[IBIS ver]   4.2
[File name]   tm4c123gh6pge_144qfp_v0p0.ibs
[File Rev]   v0p0
[Date]   Oct 16, 2013
[Source]   simulation
[Notes]   IBIS models for 144qfp package with updated GPIO models
[Disclaimer] Please be aware that in the absence of a written agreement,
   Texas Instruments (TI) assumes no liability for: 1) the
   accuracy of the IBIS models provided to your company, 2) the
   proper functioning of these IBIS models in your design or for
   any resulting applications, or; 3) infringement of patents,
   copyrights, or intellectual property rights resulting from
   your use of these IBIS models. TI provides IBIS models as a
   service to our customers and therefore reserves the right to
   limit distribution of the IBIS models.
   This preliminary model does not contain all of the possible pad
   models for each of the pad types.  The most commonly used modes
   have been provided and the next update will include all of the
   pad model combinations.
   The only missing model that needs to be highlighted is the
   model for the USB D+ and D- GPIOs.  Currently only the USB
   functionality is provided on the D+ and D- pins.  Customers
   needing to model the PGIOs associated with these pins should
   check for a newer model.
[Copyright]   Property of Texas Instruments Incorporated. Unauthorized
   reproduction and/or distribution is strictly prohibited. This
   product is protected under copyright law and trade secret law
   as an unpublished work. Copyright (C) 2013, Texas Instruments
   Incorporated, all rights reserved. These commodities are under
   the U.S. Government distribution license control. As such,
   they are not to be re-exported without the prior approval of
   the U.S. Department of Commerce.
|   Component TM4C123GH6PGE
[Component]   TM4C123GH6PGE
[Manufacturer]   Texas Instruments Inc.
[Package]
| 144-pin QFP
| variable   typ   min   max
R_Pkg   2.69E-01   2.45E-01   3.00E-01
L_pkg   7.59E-09   5.97E-09   9.02E-09
C_pkg   1.89E-12   1.71E-12   2.18E-12
[Pin]   signal_name   model_name   R_pin   L_pin   C_pin
1   PD0   GPIO8P_5V   2.98E-01   8.84E-09   1.79E-12
2   PD1   GPIO8P_5V   2.91E-01   8.75E-09   2.17E-12
3   PD2   GPIO8P_5V   2.87E-01   8.56E-09   2.13E-12
4   PD3   GPIO8P_5V   2.79E-01   8.34E-09   2.08E-12
5   VDD   POWER
6   GND   GND
7   VDDA   POWER
8   VREFAP   NC
9   VREFAM   NC
10   GNDA   GND
11   PP2   GPIO8P_5V   2.64E-01   7.47E-09   1.85E-12
12   PE3   GPIO8P_5V   2.60E-01   7.38E-09   1.83E-12
13   PE2   GPIO8P_5V   2.54E-01   7.11E-09   1.81E-12
14   PE1   GPIO8P_5V   2.53E-01   6.97E-09   1.78E-12
15   PE0   GPIO8P_5V   2.49E-01   6.94E-09   1.74E-12
16   PK0   GPIO8P_5V   2.50E-01   6.88E-09   1.72E-12
17   PK1   GPIO8P_5V   2.48E-01   6.76E-09   1.72E-12
18   PK2   GPIO8P_5V   2.48E-01   6.72E-09   1.72E-12
19   PK3   GPIO8P_5V   2.49E-01   6.89E-09   1.72E-12
20   PN2   GPIO8P_5V   2.46E-01   6.73E-09   1.72E-12
21   PH7   GPIO8P_5V   2.46E-01   6.93E-09   1.73E-12
22   PH6   GPIO8P_5V   2.45E-01   6.81E-09   1.75E-12
23   PH5   GPIO8P_5V   2.46E-01   6.87E-09   1.77E-12
24   VDD   POWER
25   GND   GND
26   PH4   GPIO8P_5V   2.52E-01   7.22E-09   1.82E-12
27   PH3   GPIO8P_5V   2.54E-01   7.29E-09   1.87E-12
28   PH2   GPIO8P_5V   2.55E-01   7.42E-09   1.92E-12
29   VDD   POWER
30   GND   GND
31   PH1   GPIO8P_5V   2.69E-01   7.93E-09   2.01E-12
32   PH0   GPIO8P_5V   2.70E-01   7.93E-09   2.06E-12
33   PC7   GPIO8P_5V   2.78E-01   8.27E-09   2.09E-12
34   PC6   GPIO8P_5V   2.85E-01   8.51E-09   2.13E-12
35   PC5   GPIO8P_5V   2.89E-01   8.59E-09   2.17E-12
36   PC4   GPIO8P_5V   2.96E-01   8.89E-09   1.79E-12
37   PA0_U0Rx   GPIO8P_5V   2.98E-01   8.92E-09   1.79E-12
38   PA1_U0Tx   GPIO8P_5V   2.94E-01   8.73E-09   2.17E-12
39   PA2_SSI0Clk   GPIO8P_5V   2.90E-01   8.64E-09   2.13E-12
40   PA3_SSI0Fss   GPIO8P_5V   2.84E-01   8.42E-09   2.10E-12
41   PA4_SSI0Rx   GPIO8P_5V   2.78E-01   8.20E-09   2.07E-12
42   PA5_SSI0Tx   GPIO8P_5V   2.75E-01   7.86E-09   2.01E-12
43   VDD   POWER
44   GND   GND
45   PA6   GPIO8P_5V   2.65E-01   7.49E-09   1.93E-12
46   PA7   GPIO8P_5V   2.65E-01   7.46E-09   1.88E-12
47   PG7   GPIO8P_5V   2.62E-01   7.29E-09   1.85E-12
48   PG6   GPIO8P_5V   2.61E-01   6.22E-09   1.80E-12
49   VDDC   POWER
50   PG5   GPIO8P_5V   2.77E-01   6.51E-09   1.82E-12
51   PG4   GPIO8P_5V   2.74E-01   7.25E-09   1.79E-12
52   PG3   GPIO8P_5V   2.72E-01   7.27E-09   1.77E-12
53   PG2   GPIO8P_5V   2.69E-01   7.15E-09   1.75E-12
54   PG1   GPIO8P_5V   2.68E-01   7.06E-09   1.74E-12
55   PG0   GPIO8P_5V   2.66E-01   7.16E-09   1.74E-12
56   VDD   POWER
57   GND   GND
58   PF7   GPIO8P_5V   2.62E-01   7.10E-09   1.77E-12
59   PF6   GPIO8P_5V   2.60E-01   7.12E-09   1.79E-12
60   PF5   GPIO8P_5V   2.60E-01   7.10E-09   1.81E-12
61   PF4   GPIO8P_5V   2.63E-01   7.31E-09   1.83E-12
62   PF0   GPIO8P_5V   2.64E-01   7.42E-09   1.86E-12
63   PF1   GPIO8P_5V   2.66E-01   7.54E-09   1.88E-12
64   PF2   GPIO8P_5V   2.67E-01   7.70E-09   1.93E-12
65   PF3   GPIO8P_5V   2.69E-01   7.70E-09   1.96E-12
66   VDD   POWER
67   GND   GND
68   PN7   GPIO8P_5V   2.80E-01   8.28E-09   2.07E-12
69   PN6   GPIO8P_5V   2.85E-01   8.41E-09   2.10E-12
70   PN5   GPIO8P_5V   2.90E-01   8.57E-09   2.13E-12
71   PN4   GPIO8P_5V   2.92E-01   8.84E-09   2.17E-12
72   WAKE_n   RST_WAKE_INPUT  2.99E-01   8.87E-09   1.79E-12
73   HIB_n   HIB_OUTPUT   2.96E-01   8.93E-09   1.79E-12
74   XOSC0   NC
75   GNDX   GND
76   XOSC1   NC
77   VBAT   POWER
78   VDD   POWER
79   GND   GND
80   PN1   GPIO8P_5V   2.66E-01   7.63E-09   1.95E-12
81   PN0   GPIO8P_5V   2.64E-01   7.60E-09   1.93E-12
82   PM7   GPIO8P_5V   2.60E-01   7.40E-09   1.88E-12
83   PM6   GPIO8P_5V   2.57E-01   7.27E-09   1.83E-12
84   PM5   GPIO8P_5V   2.60E-01   7.28E-09   1.81E-12
85   PM4   GPIO8P_5V   2.57E-01   7.18E-09   1.81E-12
86   PM3   GPIO8P_5V   2.54E-01   7.01E-09   1.78E-12
87   PM2   GPIO8P_5V   2.52E-01   6.94E-09   1.76E-12
88   PM1   GPIO8P_5V   2.51E-01   6.93E-09   1.74E-12
89   PM0   GPIO8P_5V   2.49E-01   6.90E-09   1.72E-12
90   RST_n   RST_WAKE_INPUT  2.47E-01   6.80E-09   1.71E-12
91   GND   GND
92   OSC0   NC
93   OSC1   NC
94   VDD   POWER
95   PL7   USB_PHY_DM   2.46E-01   6.82E-09   1.75E-12
96   PL6   USB_PHY_DP   2.45E-01   6.91E-09   1.78E-12
97   PB0_USB0ID   GPIO8P_5V   2.49E-01   7.12E-09   1.82E-12
98   PB1_USB0VBUS   GPIO8P_5V   2.51E-01   7.17E-09   1.84E-12
99   PB2_I2C0SCL   GPIO8P_5V   2.54E-01   7.41E-09   1.87E-12
100   PB3_I2C0SDA   GPIO8P_5V   2.57E-01   7.46E-09   1.91E-12
101   VDD   POWER
102   GND   GND
103   PL5   GPIO8P_5V   2.69E-01   7.95E-09   2.01E-12
104   PL4   GPIO8P_5V   2.72E-01   8.14E-09   2.06E-12
105   PL3   GPIO8P_5V   2.80E-01   8.31E-09   2.09E-12
106   PL2   GPIO8P_5V   2.86E-01   8.53E-09   2.13E-12
107   PL1   GPIO8P_5V   2.89E-01   8.73E-09   2.18E-12
108   PL0   GPIO8P_5V   2.97E-01   8.93E-09   1.79E-12
109   PK7   GPIO8P_5V   3.00E-01   9.02E-09   1.79E-12
110   PK6   GPIO8P_5V   2.95E-01   8.70E-09   2.17E-12
111   PK5   GPIO8P_5V   2.89E-01   8.49E-09   2.13E-12
112   PK4   GPIO8P_5V   2.82E-01   6.82E-09   2.10E-12
113   VDD   POWER
114   GND   GND
115   PC3_TDO_SWO   GPIO8P_5V   2.75E-01   6.66E-09   1.99E-12
116   PC2_TDI   GPIO8P_5V   2.71E-01   7.72E-09   1.97E-12
117   PC1_TMS_SWDIO  GPIO8P_5V   2.66E-01   7.60E-09   1.93E-12
118   PC0_TCK_SWCLK  GPIO8P_5V   2.66E-01   7.63E-09   1.88E-12
119   PN3   GPIO8P_5V   2.65E-01   7.43E-09   1.83E-12
120   PJ0   GPIO8P_5V   2.66E-01   7.34E-09   1.81E-12
121   PJ1   GPIO8P_5V   2.62E-01   7.32E-09   1.82E-12
122   PJ2   GPIO8P_5V   2.63E-01   7.29E-09   1.79E-12
123   PJ3   GPIO8P_5V   2.62E-01   6.14E-09   1.74E-12
124   VDD   POWER
125   GND   GND
126   VDDC   POWER
127   PJ4   GPIO8P_5V   2.65E-01   5.97E-09   1.74E-12
128   PJ5   GPIO8P_5V   2.62E-01   7.04E-09   1.74E-12
129   PJ6   GPIO8P_5V   2.61E-01   6.88E-09   1.75E-12
130   PJ7   GPIO8P_5V   2.60E-01   7.05E-09   1.77E-12
131   PP0   GPIO8P_5V   2.60E-01   7.07E-09   1.79E-12
132   PP1   GPIO8P_5V   2.61E-01   7.16E-09   1.81E-12
133   PE6   GPIO8P_5V   2.63E-01   7.16E-09   1.84E-12
134   PE7   GPIO8P_5V   2.65E-01   7.36E-09   1.86E-12
135   PB5   GPIO8P_5V   2.65E-01   7.51E-09   1.88E-12
136   PB4   GPIO8P_5V   2.67E-01   6.47E-09   1.93E-12
137   VDD   POWER
138   GND   GND
139   PE4   GPIO8P_5V   2.76E-01   6.72E-09   2.02E-12
140   PE5   GPIO8P_5V   2.78E-01   8.20E-09   2.07E-12
141   PD4   GPIO8P_5V   2.84E-01   8.33E-09   2.10E-12
142   PD5   GPIO8P_5V   2.90E-01   8.70E-09   2.13E-12
143   PD6   GPIO8P_5V   2.93E-01   8.73E-09   2.17E-12
144   PD7   GPIO8P_5V   3.00E-01   8.97E-09   1.79E-12
[Model Selector] GPIO8P_5V
GPIO8P_5V_I/O_2   2mA Output Buffer
GPIO8P_5V_I/O_4   4mA Output Buffer
GPIO8P_5V_I/O_8S   8mA Output Buffer with Slew Rate Control
GPIO8P_5V_I/O_8   8mA Output Buffer
GPIO8P_5V_I_WPU_2   2mA Input with Pull-Up
GPIO8P_5V_I_WPD_2   2mA Input with Pull-Down
GPIO8P_5V_I/O_OD_2   2mA Output Buffer with Open Drain
GPIO8P_5V_I/O_OD_4   4mA Output Buffer with Open Drain
GPIO8P_5V_I/O_OD_8S   8mA Output Buffer with Open Drain and Slew Rate Control
GPIO8P_5V_I/O_OD_8   8mA Output Buffer with Open Drain
[Model Selector] RST_WAKE_INPUT
RST_WAKE_IN   Input Model for the WAKE_n Pin
[Model Selector] HIB_OUTPUT
HIBERNATE_OUTPUT   Output Buffer for the HIB_n Pin
[Model Selector] USB_PHY_DP
fsdp_tx   Full Speed transmitter--12Mbps
lsdp_50pf_tx   Low speed transmitter--1.5Mbps driving 50pF cap load
lsdp_200pf_tx   Low speed transmitter--1.5Mbps driving 200pF cap load
lsdp_400pf_tx   Low speed transmitter--1.5Mbps driving 400pF cap load
lsdp_600pf_tx   Low speed transmitter--1.5Mbps driving 600pF cap load
fsdp_rx   Recieve mode--Open circuit during fs/ls recieve mode
[Model Selector] USB_PHY_DM
fsdm_tx   Full Speed transmitter--12Mbps
lsdm_50pf_tx   Low speed transmitter--1.5Mbps driving 50pF cap load
lsdm_200pf_tx   Low speed transmitter--1.5Mbps driving 200pF cap load
lsdm_400pf_tx   Low speed transmitter--1.5Mbps driving 400pF cap load
lsdm_600pf_tx 	 Low speed transmitter--1.5Mbps driving 600pF cap load
fsdm_rx   Recieve mode--Open circuit during fs/ls recieve mode
| Models and submodels in the file (24): GPIO8P_5V_I/O_2 (I/O), GPIO8P_5V_I/O_4 (I/O), GPIO8P_5V_I/O_8S (I/O), GPIO8P_5V_I/O_8 (I/O), GPIO8P_5V_I_WPU_2 (Input), GPIO8P_5V_I_WPD_2 (Input), GPIO8P_5V_I/O_OD_2 (I/O_open_drain), GPIO8P_5V_I/O_OD_4 (I/O_open_drain), GPIO8P_5V_I/O_OD_8S (I/O_open_drain), GPIO8P_5V_I/O_OD_8 (I/O_open_drain), RST_WAKE_IN (Input), HIBERNATE_OUTPUT (Output), fsdp_tx (3-state), lsdp_50pf_tx (3-state), lsdp_200pf_tx (3-state), lsdp_400pf_tx (3-state), lsdp_600pf_tx (3-state), fsdp_rx (Input), fsdm_tx (3-state), lsdm_50pf_tx (3-state), lsdm_200pf_tx (3-state), lsdm_400pf_tx (3-state), lsdm_600pf_tx (3-state), fsdm_rx (Input)
